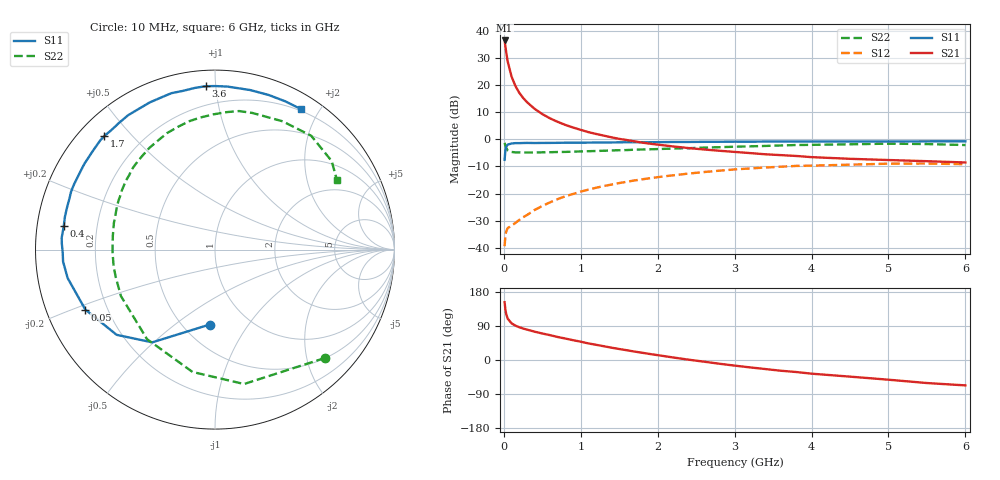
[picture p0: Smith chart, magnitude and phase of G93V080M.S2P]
! SIEMENS Small Signal Semiconductors
! BFG235
! Si NPN RF Bipolar Junction Transistor in SOT223
! VCE = 3 V  IC = 80 mA
! Common Emitter S-Parameters:  July  1994
# GHz  S  MA  R  50
!  f  S11  S21  S12  S22
! GHz  MAG  ANG  MAG  ANG  MAG  ANG  MAG  ANG
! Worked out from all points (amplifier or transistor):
!   40 points, 10 MHz to 6 GHz, reference 50 ohm
!   highest |S21| = 36.4 dB at 10 MHz (marker M1)
!   |S21| within 3 dB of that: start of sweep to 24.31 MHz
!   unconditionally stable (mu >= 1): 477.7 MHz to 1.489 GHz
!   at 200 MHz: K = 0.75, MSG = 23.4 dB, |S12| = -29.7 dB
!   at 1.5 GHz: K = 1.00, MSG = 8.1 dB, |S12| = -16.1 dB
!   at 6 GHz: K = 0.92, MSG = 0.3 dB, |S12| = -9.2 dB
!   S11 on the Smith chart (normalised r, x): 10 MHz: 0.67, -0.68; 50 MHz: 0.12, -0.22; 400 MHz: 0.08, +0.08; 1.7 GHz: 0.07, +0.42; 3.6 GHz: 0.09, +0.94; 6 GHz: 0.18, +1.76
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0.01  0.4184 -94.0  65.69 152.5  0.0108 64.5  0.8593 -44.7
0.02  0.6241 -124.1  51.59 133.6  0.017 48.3  0.7662 -77.8
0.03  0.7252 -139.1  40.55 121.7  0.0199 40.0  0.6931 -100.4
0.05  0.7961 -155.2  27 109.1  0.0232 31.8  0.6263 -127.2
0.1  0.8363 -169.1  14.27 96.8  0.0257 33.2  0.5846 -153.7
0.15  0.8491 -175.5  9.583 90.7  0.0289 38.3  0.5738 -164.6
0.2  0.8487 -179.0  7.172 86.6  0.0327 42.6  0.5724 -170.7
0.25  0.8538 177.9  5.779 83.1  0.0367 46.5  0.5703 -175.0
0.3  0.8567 175.6  4.827 80.3  0.0403 49.3  0.571 -178.6
0.4  0.8529 171.1  3.633 74.7  0.05 52.7  0.5713 176.4
0.5  0.856 167.5  2.903 69.9  0.0594 54.8  0.5745 172.2
0.6  0.857 164.4  2.426 65.6  0.0691 55.3  0.5778 168.4
0.7  0.8595 160.7  2.09 60.7  0.0794 55.1  0.5829 165.0
0.9  0.8655 155.2  1.645 52.3  0.0986 53.0  0.591 158.8
1.1  0.8678 149.0  1.352 43.7  0.1186 50.1  0.6034 152.8
1.7  0.8838 134.2  0.914 22.2  0.1749 38.5  0.6428 136.5
2.2  0.8916 122.9  0.738 6.7  0.2173 27.6  0.6745 122.8
3.2  0.9022 101.5  0.557 -19.5  0.2905 4.4  0.7401 96.4
3.6  0.912 93.2  0.511 -28.3  0.3127 -5.6  0.7686 85.2
4.5  0.9103 77.6  0.437 -43.9  0.3407 -25.4  0.808 62.2
5.5  0.9143 64.6  0.395 -60.8  0.3581 -47.2  0.8161 37.2
6  0.9174 58.7  0.374 -67.0  0.3479 -55.4  0.7827 29.9
